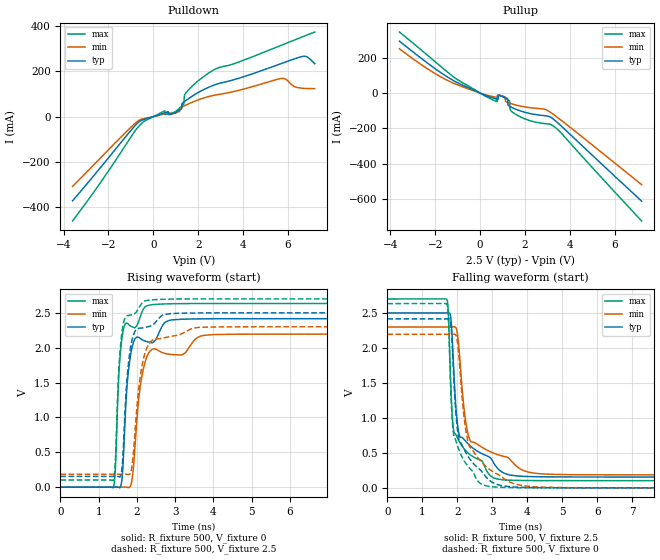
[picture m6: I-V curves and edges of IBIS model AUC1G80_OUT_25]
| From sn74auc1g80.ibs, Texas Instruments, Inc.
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[Model]   AUC1G80_OUT_25
Model_type  Output
Vref =   0
Rref =   500
Cref =   30p
Vmeas =   1.25
| variable   typ   min   max
C_comp   7.88pF   0.10pF   24.69pF
| C_pullup   8.73pF   0.10pF   24.69pF
| C_pulldown   7.03pF   1.88pF   16.28pF
[Temperature Range]   40   100   -40
| Ambient temperature   25   85   -40
[Voltage range]   2.5   2.3   2.7
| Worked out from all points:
|   slope of the pulldown table from 0 to 0.375 V, typ, clamps not added: 30.9 ohm
|   slope of the pullup table from 0 to 0.375 V, typ, clamps not added: 19.1 ohm
|   rising waveform, R_fixture 500, V_fixture 0: 20-80 % time 194ps typ, 265ps min, 147ps max; typ from 0 V to 2.42 V
|   falling waveform, R_fixture 500, V_fixture 2.5: 20-80 % time 455ps typ, 553ps min, 338ps max; typ from 2.5 V to 0.154 V
|   rising waveform, R_fixture 500, V_fixture 2.5: 20-80 % time 193ps typ, 263ps min, 145ps max; typ from 0.154 V to 2.5 V
|   falling waveform, R_fixture 500, V_fixture 0: 20-80 % time 402ps typ, 510ps min, 291ps max; typ from 2.42 V to 0 V
[Pulldown]
| AUC1G80_OUT_25
|   Voltage   I(typ)   I(min)   I(max)
-3.6V     -372.5mA   -309mA     -462.1mA
-460mV    -13.88mA   -9.419mA   -24.18mA
515mV     17.09mA    12.69mA    26.01mA
995mV     19.39mA    16.37mA    22.93mA
1.265V    34.6mA     42.17mA    46.77mA
1.365V    64.98mA    47.02mA    56.26mA
1.4V      67.51mA    48.7mA     96.65mA
1.565V    79.22mA    56.41mA    117.9mA
2.705V    139.7mA    94.6mA     207.5mA
5.68V     234.2mA    168.7mA    315.1mA
6.74V     267.5mA    125.2mA    356.8mA
7.2V      234.4mA    124.1mA    374.7mA
[Pullup]
| AUC1G80_OUT_25
|   Voltage   I(typ)   I(min)   I(max)
-3.6V     293.6mA    250.6mA    345.6mA
-980mV    56.7mA     45.13mA    73.07mA
745mV     -34.33mA   -24.78mA   -47.94mA
770mV     -35.18mA   -25.36mA   -13.1mA
1.065V    -22.79mA   -19.92mA   -25.37mA
1.22V     -31.46mA   -52.78mA   -37.36mA
1.235V    -65.07mA   -53.46mA   -38.52mA
1.305V    -74.54mA   -56.59mA   -44.02mA
1.36V     -78.26mA   -58.92mA   -98.77mA
1.815V    -102mA     -74.28mA   -135.8mA
3.31V     -151.9mA   -125.1mA   -190.9mA
7.2V      -611.9mA   -518.4mA   -724.2mA
[Ramp]
| AUC1G80_OUT_25
| variable   typ   min   max
dV/dt_r   1.46/1.95E-10   1.32/2.65E-10   1.59/1.48E-10
dV/dt_f   1.41/4.55E-10   1.27/5.51E-10   1.56/3.38E-10
R_load = 500
[Rising Waveform]
| AUC1G80_OUT_25
R_fixture =   500
C_fixture =   0
L_fixture =   0
V_fixture =   0
V_fixture_min = 0
V_fixture_max = 0
|   Time   V(typ)   V(min)   V(max)
0s        10.1nV     29.66nV    1.873nV
1.38ns    128.6uV    -2.457uV   -4.709mV
1.435ns   287.3uV    -76.78nV   253.5mV
1.535ns   -5.269mV   69uV       1.685V
1.64ns    352.3mV    402.3uV    2.244V
1.74ns    1.434V     -736.9uV   2.35V
1.865ns   1.986V     82.03mV    2.303V
2.08ns    2.138V     1.412V     2.432V
2.305ns   2.081V     1.922V     2.608V
21.22ns   2.416V     2.195V     2.634V
[Falling Waveform]
| AUC1G80_OUT_25
R_fixture =   500
C_fixture =   0
L_fixture =   0
V_fixture =   2.5
V_fixture_min = 2.3
V_fixture_max = 2.7
|   Time   V(typ)   V(min)   V(max)
0s        2.5V       2.3V       2.7V
1.705ns   2.5V       2.3V       2.686V
1.745ns   2.501V     2.3V       2.505V
1.82ns    2.406V     2.3V       1.404V
1.91ns    1.578V     2.302V     785mV
2.055ns   760mV      1.96V      666.6mV
2.345ns   612.5mV    707.3mV    482.2mV
3.14ns    285.8mV    477.9mV    126.9mV
4.685ns   156.5mV    193.3mV    103.2mV
21.22ns   154.5mV    185.7mV    102.7mV
[Rising Waveform]
| AUC1G80_OUT_25
R_fixture =   500
C_fixture =   0
L_fixture =   0
V_fixture =   2.5
V_fixture_min = 2.3
V_fixture_max = 2.7
|   Time   V(typ)   V(min)   V(max)
0s        154.5mV    185.7mV    102.6mV
1.38ns    154.6mV    185.7mV    98.08mV
1.435ns   154.7mV    185.7mV    358mV
1.535ns   149.4mV    185.7mV    1.761V
1.635ns   462.7mV    186mV      2.314V
1.735ns   1.514V     185.5mV    2.457V
1.845ns   2.037V     223.3mV    2.47V
2.06ns    2.279V     1.473V     2.58V
2.25ns    2.296V     1.984V     2.677V
21.22ns   2.5V       2.3V       2.7V
[Falling Waveform]
| AUC1G80_OUT_25
R_fixture =   500
C_fixture =   0
L_fixture =   0
V_fixture =   0
V_fixture_min = 0
V_fixture_max = 0
|   Time   V(typ)   V(min)   V(max)
0s        2.416V     2.195V     2.634V
1.71ns    2.416V     2.195V     2.615V
1.75ns    2.417V     2.195V     2.377V
1.815ns   2.34V      2.195V     1.402V
1.905ns   1.534V     2.197V     738.6mV
2.04ns    712mV      1.926V     552.4mV
2.305ns   453.8mV    666.4mV    310.7mV
2.82ns    156.4mV    305.4mV    29.49mV
4.5ns     2.076mV    8.644mV    563.4uV
21.22ns   24.64uV    4.407uV    11.15uV
